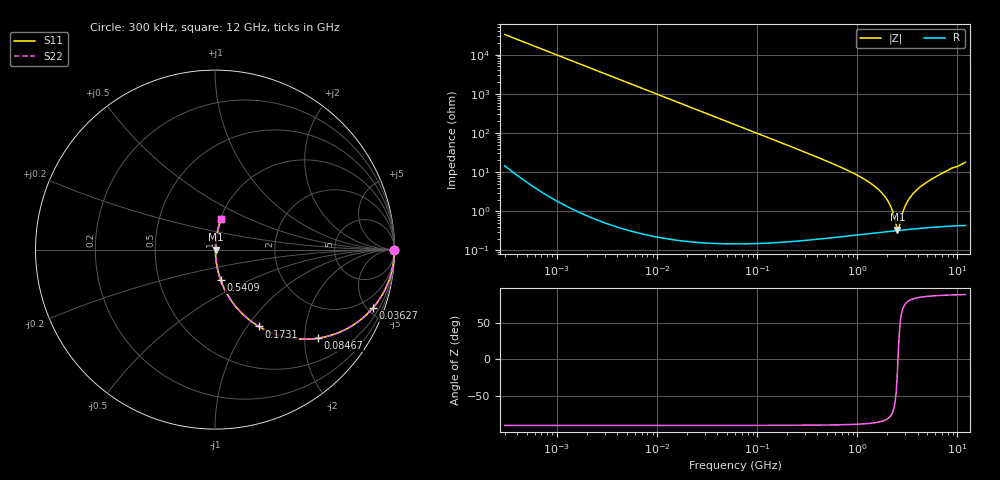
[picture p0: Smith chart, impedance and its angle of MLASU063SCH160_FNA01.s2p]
! MLASU063SCH160_FNA01  S-PARAMETER MODEL  ( Standard Model )
! Model Generated by TAIYO YUDEN Corporation (http://www.ty-top.com)
! Version 1.0
! TAIYO YUDEN Control No. 240819
! Copyright(c) 2024 TAIYO YUDEN CO.,LTD. All Rights Reserved.
! Product Description (link to TY-COMPAS)
! https://ds.yuden.co.jp/TYCOMPAS/or/detail?pn=MLASU063SCH160JFNA01&u=M
! Products Name : Multilayer Ceramic Capacitors
! Characteristics :
!  Capacitance : 16 [pF] , Rated Voltage : 50 [V] , TCC : CH / C0H
!  Case Size : 0.6 x 0.3 / 0.024 x 0.012 [mm/inch] , Thickness : 0.3 / 0.012 [mm/inch]
!  (Conditions: Temperature = 25 [degC] , DC Bias Voltage = 0 [V])
! External Node Assignments :
!  1  o---| |---o  2
! GND o---------o GND
! Frequency Range : 0.3MHz  -  12000MHz  [ 401 STEP ]
# MHZ S RI R 50
! Freq[MHz].  S11 Real  S11 Imag  S21 Real  S21 Imag  S12 Real  S12 Imag  S22 Real  S22 Imag
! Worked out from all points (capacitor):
!   401 points, 300 kHz to 12 GHz, reference 50 ohm
!   read as one part in series: C = 16.1 pF near 316.3 kHz
!   lowest |Z| = 338 mohm at 2.514 GHz (marker M1)
!   series resonance near 2.546 GHz, so ESL is about 240 pH
!   S11 on the Smith chart (normalised r, x): 300 kHz: open; 36.27 MHz: 1.00, -5.43; 84.67 MHz: 1.00, -2.33; 173.1 MHz: 1.00, -1.13; 540.9 MHz: 1.00, -0.35; 12 GHz: 1.01, +0.36
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0.3  1 -0.00304  1.06e-05 0.00304  1.06e-05 0.00304  1 -0.00304
1.769972  0.9997 -0.018  0.000325 0.018  0.000325 0.018  0.9997 -0.018
10.44266  0.9889 -0.1048  0.0111 0.1048  0.0111 0.1048  0.9889 -0.1048
36.27049  0.8806 -0.324  0.1194 0.324  0.1194 0.324  0.8806 -0.324
60  0.7293 -0.4439  0.2707 0.4439  0.2707 0.4439  0.7293 -0.4439
84.66778  0.5748 -0.4937  0.4252 0.4937  0.4252 0.4937  0.5748 -0.4937
173.124  0.2437 -0.4279  0.7563 0.4279  0.7563 0.4279  0.2437 -0.4279
353.9943  0.0709 -0.2532  0.9291 0.2532  0.9291 0.2532  0.0709 -0.2532
540.8523  0.0313 -0.1682  0.9687 0.1682  0.9687 0.1682  0.0313 -0.1682
943.3804  0.0104 -0.089  0.9896 0.089  0.9896 0.089  0.0104 -0.089
1366.97  0.00532 -0.0509  0.9947 0.0509  0.9947 0.0509  0.00532 -0.0509
1781.601  0.00372 -0.0281  0.9963 0.0281  0.9963 0.0281  0.00372 -0.0281
2088.533  0.0033 -0.0154  0.9967 0.0154  0.9967 0.0154  0.0033 -0.0154
2261.293  0.00321 -0.00916  0.9968 0.00916  0.9968 0.00916  0.00321 -0.00916
2448.343  0.0032 -0.00303  0.9968 0.00303  0.9968 0.00303  0.0032 -0.00303
2514.07  0.00322 -0.000989  0.9968 0.000989  0.9968 0.000989  0.00322 -0.000989
2650.866  0.00327 0.00317  0.9967 -0.00317  0.9967 -0.00317  0.00327 0.00317
2870.14  0.00342 0.00946  0.9966 -0.00946  0.9966 -0.00946  0.00342 0.00946
3107.553  0.00365 0.0158  0.9964 -0.0158  0.9964 -0.0158  0.00365 0.0158
3944.255  0.00484 0.0351  0.9952 -0.0351  0.9952 -0.0351  0.00484 0.0351
6354.153  0.0105 0.0804  0.9895 -0.0804  0.9895 -0.0804  0.0105 0.0804
12000  0.0348 0.1716  0.9652 -0.1716  0.9652 -0.1716  0.0348 0.1716
